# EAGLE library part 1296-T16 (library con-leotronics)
1.27mm SINGLE ROW FEMALE SOCKET Source: http://www.leotronics.co.uk/Conexcon/Data%20Sheets/sec.%20A/1296ing.pdf
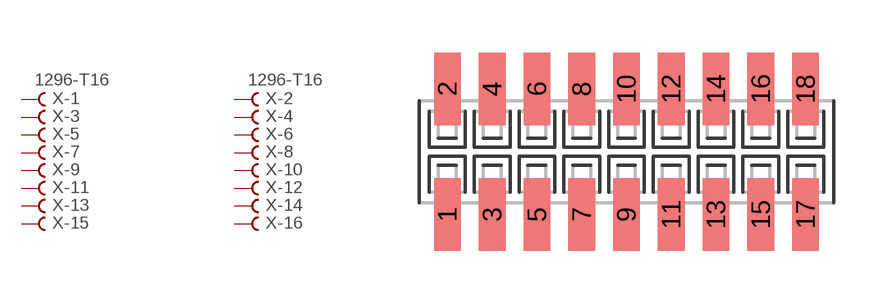
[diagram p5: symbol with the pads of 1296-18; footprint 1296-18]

Designator prefix X; gates -1=FVAL -2=FVAL -3=F -4=F -5=F -6=F -7=F -8=F -9=F -10=F -11=F -12=F -13=F -14=F -15=F -16=F -17=F -18=F

## 1296-T16 (OC_FARNELL: unknown; OC_NEWARK: unknown)  [1296-18]
1  -1:B  pas
2  -2:B  pas
3  -3:B  pas
4  -4:B  pas
5  -5:B  pas
6  -6:B  pas
7  -7:B  pas
8  -8:B  pas
9  -9:B  pas
10  -10:B  pas
11  -11:B  pas
12  -12:B  pas
13  -13:B  pas
14  -14:B  pas
15  -15:B  pas
16  -16:B  pas
17  -17:B  pas
18  -18:B  pas

## Footprint 1296-18 (pad centres in mm)
1.27mm SINGLE ROW FEMALE SOCKET Source: http://www.leotronics.co.uk/Conexcon/Data%20Sheets/sec.%20A/1296ing.pdf
smd 0.76 x 2.05: 1 -5.08,-1.78; 2 -5.08,1.78; 3 -3.81,-1.78; 4 -3.81,1.78; 5 -2.54,-1.78; 6 -2.54,1.78; 7 -1.27,-1.78; 8 -1.27,1.78; 9 0,-1.78; 10 0,1.78; 11 1.27,-1.78; 12 1.27,1.78; 13 2.54,-1.78; 14 2.54,1.78; 15 3.81,-1.78; 16 3.81,1.78; 17 5.08,-1.78; 18 5.08,1.78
